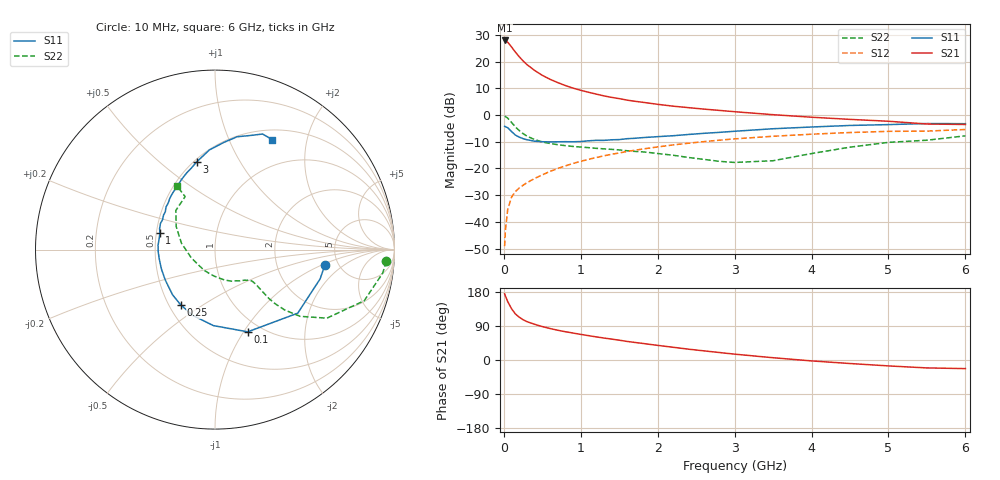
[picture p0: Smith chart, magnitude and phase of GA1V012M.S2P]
! Infineon Technologies  Discrete & RF Semiconductors
! BF775
! Si NPN RF Bipolar Junction Transistor in SOT23
! VCE = 1 V  IC = 12 mA
! Common Emitter S-Parameters:  May  1996
# GHz  S  MA  R  50
!  f  S11  S21  S12  S22
! GHz  MAG  ANG  MAG  ANG  MAG  ANG  MAG  ANG
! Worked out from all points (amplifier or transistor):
!   36 points, 10 MHz to 6 GHz, reference 50 ohm
!   highest |S21| = 28.0 dB at 10 MHz (marker M1)
!   |S21| within 3 dB of that: start of sweep to 114.8 MHz
!   unconditionally stable (mu >= 1): 409.9 MHz to end of sweep
!   at 250 MHz: K = 0.80, MSG = 23.3 dB, |S12| = -26.3 dB
!   at 1.4 GHz: K = 1.17, MAG = 8.1 dB, |S12| = -14.7 dB
!   at 6 GHz: K = 1.04, MAG = -0.2 dB, |S12| = -5.4 dB
!   S11 on the Smith chart (normalised r, x): 10 MHz: 3.90, -1.10; 100 MHz: 0.86, -1.04; 250 MHz: 0.57, -0.41; 1 GHz: 0.52, +0.11; 3 GHz: 0.52, +0.67; 6 GHz: 0.62, +1.46
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0.01  0.6179 -8.1  25.11 174.6  0.0035 86.2  0.9572 -3.9
0.02  0.6079 -15.6  24.91 169.0  0.0069 80.3  0.9432 -8.0
0.05  0.5814 -37.5  23.22 154.3  0.0169 73.4  0.879 -18.9
0.1  0.4931 -68.3  18.99 135.3  0.0291 64.7  0.7312 -31.5
0.15  0.4235 -91.2  15.18 121.6  0.0369 59.9  0.6024 -38.1
0.2  0.3873 -108.4  12.44 112.9  0.043 58.7  0.5141 -40.9
0.25  0.3624 -121.8  10.36 106.3  0.0485 58.7  0.4504 -42.0
0.3  0.3455 -133.1  8.87 101.3  0.0541 59.7  0.4049 -42.2
0.4  0.3249 -148.4  6.888 94.2  0.065 61.0  0.3485 -41.4
0.5  0.3176 -159.9  5.573 88.2  0.0759 62.3  0.3147 -40.7
0.6  0.3148 -169.8  4.703 83.1  0.0883 63.0  0.2946 -40.3
0.7  0.3166 -177.6  4.076 78.6  0.0999 63.3  0.2793 -40.3
0.8  0.3181 175.7  3.585 74.6  0.1118 63.0  0.2679 -40.6
1  0.3202 163.5  2.921 67.6  0.1362 62.1  0.2523 -42.4
1.1  0.3302 159.2  2.685 64.3  0.1485 61.2  0.2458 -44.1
1.6  0.3618 139.0  1.914 49.1  0.2079 56.4  0.2153 -53.9
2.2  0.4111 120.7  1.473 33.6  0.2765 48.8  0.1772 -72.7
3  0.4988 101.9  1.159 15.4  0.3591 37.5  0.1298 -119.2
3.5  0.5562 93.2  1.02 6.0  0.4017 30.3  0.1398 -160.6
4.5  0.6407 78.9  0.833 -9.3  0.4719 16.4  0.2511 149.4
5.5  0.6965 67.6  0.682 -20.9  0.5018 2.6  0.3387 119.4
6  0.6907 62.6  0.668 -22.7  0.5379 -1.3  0.4094 120.8
